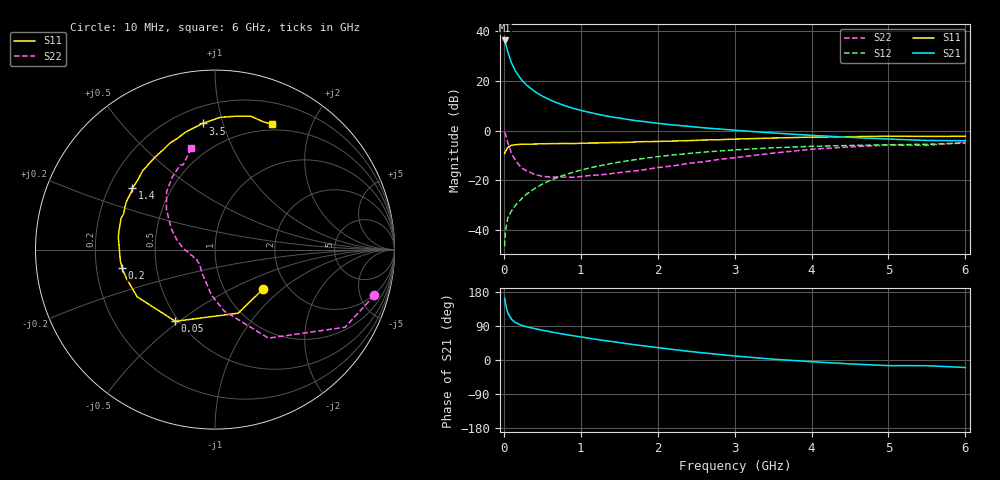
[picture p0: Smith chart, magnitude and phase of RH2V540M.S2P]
! SIEMENS Small Signal Semiconductors
! BFR106
! Si NPN RF Bipolar Junction Transistor in SOT23
! VCE = 2.5 V  IC = 40 mA
! Common Emitter S-Parameters:  August  1996
# GHz  S  MA  R  50
!  f  S11  S21  S12  S22
! GHz  MAG  ANG  MAG  ANG  MAG  ANG  MAG  ANG
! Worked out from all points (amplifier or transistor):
!   36 points, 10 MHz to 6 GHz, reference 50 ohm
!   highest |S21| = 36.1 dB at 10 MHz (marker M1)
!   |S21| within 3 dB of that: start of sweep to 38.04 MHz
!   unconditionally stable (mu >= 1): 251.2 MHz to 2.509 GHz; 5.312 GHz to end of sweep
!   at 250 MHz: K = 1.00, MSG = 23.2 dB, |S12| = -26.8 dB
!   at 1.4 GHz: K = 1.06, MAG = 7.8 dB, |S12| = -13.2 dB
!   at 6 GHz: K = 1.00, MAG = 0.3 dB, |S12| = -5.1 dB
!   S11 on the Smith chart (normalised r, x): 10 MHz: 1.51, -0.75; 50 MHz: 0.48, -0.48; 200 MHz: 0.31, -0.09; 1.4 GHz: 0.30, +0.30; 3.5 GHz: 0.31, +0.86; 6 GHz: 0.43, +1.47
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0.01  0.3466 -39.1  63.93 163.4  0.0048 80.4  0.9238 -16.0
0.02  0.3771 -70.0  57.66 150.3  0.0092 69.3  0.844 -30.8
0.05  0.4567 -119.0  38.55 124.8  0.0175 59.1  0.5761 -58.9
0.1  0.5072 -148.8  22.68 107.4  0.0246 58.6  0.3466 -81.4
0.15  0.518 -161.6  15.63 98.9  0.0315 61.6  0.2535 -94.7
0.2  0.5281 -168.6  11.97 94.1  0.0385 64.3  0.2009 -102.5
0.25  0.531 -173.4  9.591 90.2  0.0458 66.4  0.1698 -111.0
0.3  0.5313 -176.8  8.041 87.5  0.0536 68.3  0.1547 -116.7
0.4  0.5355 177.2  6.091 82.9  0.0686 69.5  0.1321 -127.1
0.5  0.543 172.7  4.896 78.6  0.0841 69.6  0.1206 -134.4
0.6  0.5452 169.0  4.106 74.7  0.0994 69.4  0.1171 -139.4
0.7  0.5474 164.9  3.548 70.8  0.1147 68.7  0.1172 -144.7
0.9  0.547 158.6  2.793 64.1  0.1453 66.6  0.1153 -153.4
1.1  0.5608 151.8  2.332 57.7  0.1751 64.0  0.1246 -158.9
1.4  0.5745 143.4  1.873 49.0  0.2185 59.5  0.137 -167.2
1.7  0.5886 134.7  1.592 40.3  0.2597 54.9  0.1551 -176.0
2.2  0.615 122.6  1.293 27.8  0.3237 46.8  0.1956 171.4
2.8  0.6542 108.6  1.073 14.7  0.3889 37.1  0.2635 155.6
3.5  0.7062 95.6  0.893 2.2  0.4508 26.3  0.3524 140.2
4.5  0.7523 81.0  0.73 -10.3  0.5015 11.8  0.4692 120.5
5.5  0.7613 69.4  0.632 -15.1  0.5309 2.7  0.5042 110.7
6  0.7667 65.4  0.624 -19.8  0.559 -4.2  0.5824 103.0
